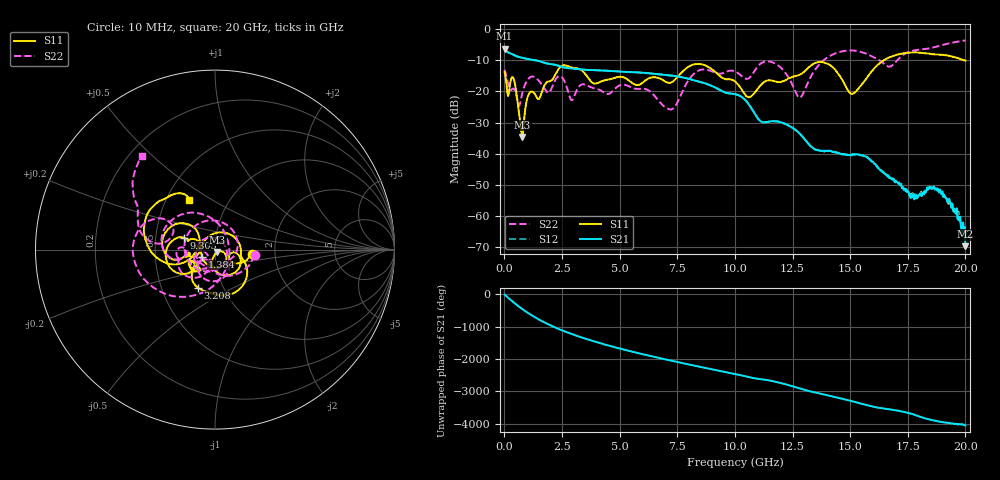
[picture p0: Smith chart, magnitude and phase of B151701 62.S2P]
!  2-Port S-parameters saved by WinCal
! VAR MeasName=S-Parameters (CALIBRATED_DATA) read from VNA (N5244A)
! VAR MeasDate=2015-12-24 19:17:19
! VAR NAME=B151701 62
! VAR FILENAME=B151701 62.S2P
! VAR DATE=2015-12-24 19:17:19
! VAR PHYS_PORTS=1,3
# Hz S DB R 50
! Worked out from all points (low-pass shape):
!   801 points, 10 MHz to 20 GHz, reference 50 ohm
!   highest |S21| = -6.24 dB at 10 MHz (marker M1); lowest = -69.8 dB at 20 GHz (marker M2)
!   |S21| within 3 dB of the highest: start of sweep to 825.2 MHz
!   lowest |S11| = -34.7 dB at 784.6 MHz (marker M3), VSWR 1.04, Z = 51.3 - j1.39 ohm
!   |S11| at or under -10 dB: start of sweep to 16.45 GHz; 19.96917 GHz to end of sweep
!   |S22| runs from -25.8 to -3.6 dB; largest |S21 - S12| = 0.0011
!   S11 on the Smith chart (normalised r, x): 10 MHz: 1.51, -0.07; 1.384 GHz: 0.86, -0.07; 3.208 GHz: 0.76, -0.34; 9.305 GHz: 0.70, +0.09; 20 GHz: 0.65, +0.40
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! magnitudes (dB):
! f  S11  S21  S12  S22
! 10 MHz  -13.8  -6.2  -6.2  -13.0
! 409.8 MHz  -16.1  -8.3  -8.3  -19.1
! 784.6 MHz  -34.7  -9.2  -9.2  -20.3
! 1.059 GHz  -20.8  -9.6  -9.6  -15.8
! 1.384 GHz  -21.6  -10.0  -10.0  -15.8
! 2.484 GHz  -11.8  -12.1  -12.0  -15.3
! 2.909 GHz  -12.3  -12.6  -12.6  -22.8
! 3.208 GHz  -12.6  -12.8  -12.8  -18.7
! 3.358 GHz  -13.2  -13.0  -12.9  -17.8
! 6.682 GHz  -15.7  -14.5  -14.5  -22.9
! 7.281 GHz  -17.0  -14.9  -14.9  -25.6
! 8.281 GHz  -11.2  -16.5  -16.5  -13.9
! 9.305 GHz  -14.7  -19.4  -19.3  -14.3
! 10.01 GHz  -16.8  -20.9  -20.9  -13.5
! 10.6 GHz  -21.9  -24.2  -24.1  -15.8
! 11.63 GHz  -16.5  -29.6  -29.6  -10.6
! 12.8 GHz  -14.7  -33.6  -33.5  -22.0
! 13.35 GHz  -11.4  -38.0  -38.1  -14.4
! 15.1 GHz  -20.8  -40.3  -40.5  -6.8
! 16.68 GHz  -9.1  -47.8  -47.5  -12.0
! 18.9 GHz  -8.2  -51.6  -52.1  -5.3
! 20 GHz  -10.1  -69.8  -66.2  -3.6
